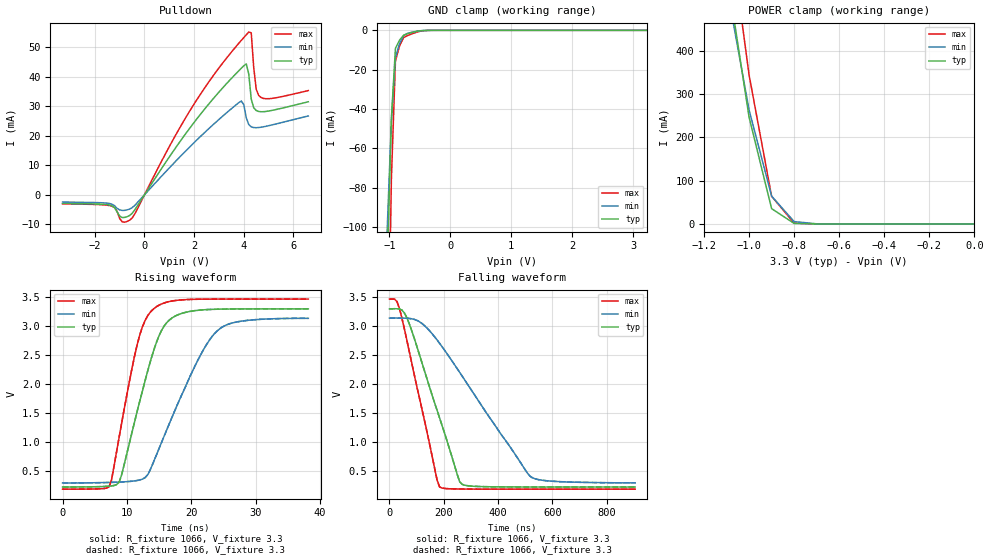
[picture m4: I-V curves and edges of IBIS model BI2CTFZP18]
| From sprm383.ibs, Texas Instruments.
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|   Model BI2CTFZP18
[Model]   BI2CTFZP18
Model_type   I/O_open_drain
Polarity   Non-Inverting
Enable   Active-Low
Vinl =  0.99
Vinh =  2.31
Cref =  400pF
Rref =  1.066k
Vref =  1.8V
Vmeas =  1.65
C_comp   1.30605p   1.212672p   1.4178p
[Model Spec]
Vinl   0.99   0.942   1.041
Vinh   2.31   2.198   2.429
[Temperature Range]   25   105   0
[Voltage Range]   3.3   3.14   3.47
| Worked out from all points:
|   slope of the pulldown table from 0 to 0.495 V, typ, clamps not added: 76.9 ohm
|   GND clamp passes 1 mA (typ) near -0.62 V on its own axis
|   POWER clamp passes 1 mA (typ) near -0.78 V on its own axis
|   rising waveform, R_fixture 1066, V_fixture 3.3: 20-80 % time 4.4ns typ, 6.87ns min, 3.5ns max; typ from 0.221 V to 3.3 V
|   rising waveform, R_fixture 1066, V_fixture 3.3: 20-80 % time 4.4ns typ, 6.87ns min, 3.5ns max; typ from 0.221 V to 3.3 V
|   falling waveform, R_fixture 1066, V_fixture 3.3: 20-80 % time 125ns typ, 247ns min, 91.7ns max; typ from 3.3 V to 0.221 V
|   falling waveform, R_fixture 1066, V_fixture 3.3: 20-80 % time 125ns typ, 247ns min, 91.7ns max; typ from 3.3 V to 0.221 V
[POWER_clamp]
|   voltage   I(typ)   I(min)   I(max)
-3.3V     9.936A     8.589A     10.91A
-1.067V   472.1mA    454mA      603.1mA
-1.033V   359.2mA    358.5mA    473.4mA
-1V       246.3mA    263mA      343.7mA
-900mV    35.32mA    64.26mA    63.74mA
-800mV    1.172mA    5.429mA    1.89mA
-700mV    29.29uA    327uA      33.79uA
-11.55fV  40.21nA    28.69nA    188.6nA
[Pulldown]
|   voltage   I(typ)   I(min)   I(max)
-3.3V     -2.959mA   -2.465mA   -3.074mA
-1.4V     -3.494mA   -2.969mA   -3.666mA
-500mV    -6.316mA   -4.377mA   -7.884mA
1.8V      22.32mA    16.03mA    28.1mA
3.8V      42.06mA    31.26mA    51.39mA
4V        43.74mA    30.57mA    53.32mA
4.1V      44.39mA    26.1mA     54.26mA
4.2V      40.99mA    23.82mA    55.17mA
4.3V      32.42mA    23.04mA    54.92mA
4.5V      28.58mA    22.74mA    35.78mA
4.6V      28.25mA    22.8mA     33.7mA
6.6V      31.54mA    26.73mA    35.34mA
[GND_clamp]
|   voltage   I(typ)   I(min)   I(max)
-3.3V     -13.47A    -11.59A    -14.63A
-1.033V   -119.7mA   -99.68mA   -199.4mA
-966.7mV  -45.02mA   -45.95mA   -75.71mA
-900mV    -9.123mA   -13.9mA    -15.56mA
-833.3mV  -5.01mA    -6.704mA   -8.034mA
-766.7mV  -2.541mA   -2.574mA   -3.727mA
-700mV    -1.716mA   -1.51mA    -2.64mA
-500mV    -222.4uA   -256.4uA   -486.2uA
-300mV    -1.786uA   -4.305uA   -6.617uA
3.233V    39.65nA    29.25nA    179.4nA
[Ramp]
| variable   typ   min   max
dV/dt_f   1.855813/0.1258291u   1.714978/0.2475095u   1.9833/92.22418n
dV/dt_r  22.53978m/1.173597n   15.02792m/2.17215n   25.55377m/0.8787091n
R_load = 1.066k
[Rising Waveform]
R_fixture = 1066
V_fixture = 3.3
V_fixture_min = 3.14
V_fixture_max = 3.47
|   time   V(typ)   V(min)   V(max)
0s        220.8mV    289.7mV    183.5mV
7.2ns     234.5mV    299mV      220mV
8.8ns     304.2mV    305mV      1.085V
11.6ns    1.529V     333mV      2.682V
12.8ns    2.047V     379.9mV    3.093V
14.2ns    2.594V     668.8mV    3.305V
17ns      3.142V     1.424V     3.436V
21.4ns    3.279V     2.492V     3.467V
24ns      3.294V     2.915V     3.469V
38.2ns    3.3V       3.137V     3.47V
[Rising Waveform]
R_fixture = 1066
V_fixture = 3.3
V_fixture_min = 3.14
V_fixture_max = 3.47
|   time   V(typ)   V(min)   V(max)
0s        220.8mV    289.7mV    183.5mV
7.2ns     234.5mV    299mV      220mV
8.8ns     304.2mV    305mV      1.085V
11.6ns    1.529V     333mV      2.682V
12.8ns    2.047V     379.9mV    3.093V
14.2ns    2.594V     668.8mV    3.305V
17ns      3.142V     1.424V     3.436V
21.4ns    3.279V     2.492V     3.467V
24ns      3.294V     2.915V     3.469V
38.2ns    3.3V       3.137V     3.47V
[Falling Waveform]
R_fixture = 1066
V_fixture = 3.3
V_fixture_min = 3.14
V_fixture_max = 3.47
|   time   V(typ)   V(min)   V(max)
0s        3.3V       3.14V      3.47V
27.6ns    3.302V     3.141V     3.428V
64.4ns    3.143V     3.138V     2.752V
119.8ns   2.368V     3.047V     1.564V
175.2ns   1.55V      2.764V     343.9mV
184.6ns   1.414V     2.705V     221.6mV
258.4ns   313.4mV    2.203V     186.3mV
267.6ns   267.6mV    2.138V     185.8mV
517ns     221mV      410.4mV    183.5mV
904.8ns   220.8mV    292.9mV    183.5mV
[Falling Waveform]
R_fixture = 1066
V_fixture = 3.3
V_fixture_min = 3.14
V_fixture_max = 3.47
|   time   V(typ)   V(min)   V(max)
0s        3.3V       3.14V      3.47V
27.6ns    3.302V     3.141V     3.428V
64.4ns    3.143V     3.138V     2.752V
119.8ns   2.368V     3.047V     1.564V
175.2ns   1.55V      2.764V     343.9mV
184.6ns   1.414V     2.705V     221.6mV
258.4ns   313.4mV    2.203V     186.3mV
267.6ns   267.6mV    2.138V     185.8mV
517ns     221mV      410.4mV    183.5mV
904.8ns   220.8mV    292.9mV    183.5mV
